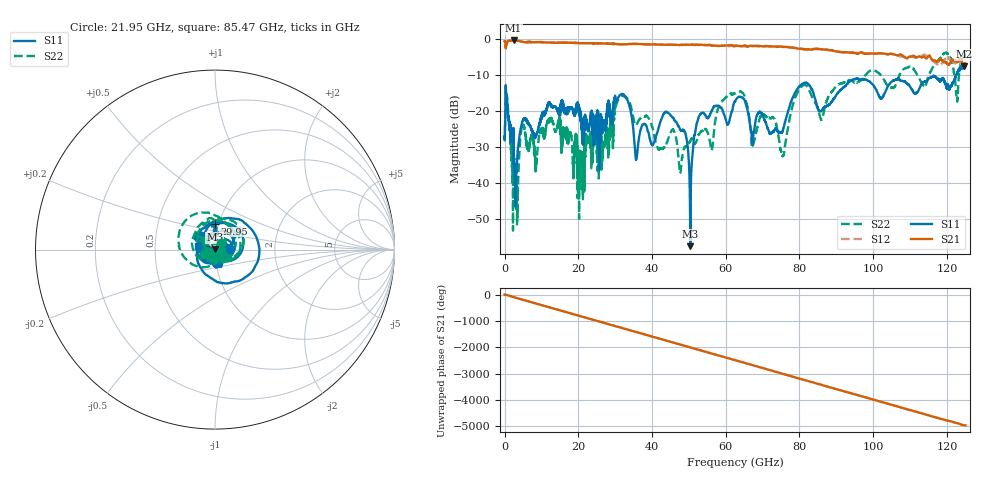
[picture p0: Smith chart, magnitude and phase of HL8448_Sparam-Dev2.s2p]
! 7/28/2025 10:33:41 AM
! H:\PROTOTYPE_DATA\110GHZ - KELVIN BT\7-28-25\4378.S2P
! CHANNEL.1
! TR.MEASUREMENT
! CORRECTED.DATA
! RF.CORRECTION: FULL.TWO.PORT.CAL.PORT.1.2
! AVERAGING: 1 PointByPoint
! IF.BANDWIDTH: 1KHZ
! SWEEPTYPE:  FREQ.SWEEP(Linear)
! Reference Plane Port Info
! PORT:  PORT1  PORT2
! DISTANCE:  0  m  0  m
! TIME:  0  s  0  s
! PHASE.OFFSET:  0 °  0 °
! LOSS:  0  dB  0  dB
! REF.LOSS:  0  dB  0  dB
! REF.FREQ:  0  Hz  0  Hz
! Power Info
! POWER:  -10  dBm  -10  dBm
! EFF.POWER:  -10  dBm  -10  dBm
! POWER(>54G):  -10  dBm  -10  dBm
! EFF.POWER(>54G):  -10  dBm  -10  dBm
! SOURCE.ATTEN:  0  dB  0  dB
! TEST.ATTEN:  0  dB  0  dB
# GHZ S RI R 50.0
! FREQ.GHZ  S11RE  S11IM  S21RE  S21IM  S12RE  S12IM  S22RE  S22IM
!; PortSelection: Port_12
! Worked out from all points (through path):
!   5000 points, 25 MHz to 125 GHz, reference 50 ohm
!   highest |S21| = -0.36 dB at 2.45 GHz (marker M1); lowest = -7.5 dB at 124.6 GHz (marker M2)
!   group delay of S21, straight-line fit = 111 ps
!   lowest |S11| = -57.7 dB at 50.4 GHz (marker M3), VSWR 1.00, Z = 49.9 + j0.101 ohm
!   |S11| at or under -10 dB: start of sweep to 122.5 GHz
!   |S22| runs from -53.3 to -3.8 dB; largest |S21 - S12| = 0.13
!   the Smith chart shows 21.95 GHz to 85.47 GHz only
!   S11 on the Smith chart (normalised r, x): 21.95 GHz: 1.18, +0.01; 29.95 GHz: 0.95, +0.28; 85.47 GHz: 0.82, +0.03
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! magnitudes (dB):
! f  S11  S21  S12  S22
! 25 MHz  -27.1  -0.6  -0.5  -27.3
! 875 MHz  -19.5  -0.6  -0.6  -18.7
! 2.45 GHz  -25.0  -0.4  -0.4  -27.1
! 12.38 GHz  -17.9  -0.9  -0.9  -23.0
! 20.88 GHz  -23.7  -1.1  -1.1  -32.7
! 21.95 GHz  -21.8  -1.1  -1.1  -26.4
! 29.95 GHz  -16.8  -1.3  -1.4  -19.6
! 33.27 GHz  -16.8  -1.4  -1.4  -16.5
! 35.75 GHz  -33.5  -1.3  -1.3  -23.9
! 41.7 GHz  -25.1  -1.5  -1.5  -30.5
! 48.7 GHz  -25.5  -1.6  -1.6  -30.4
! 50.4 GHz  -57.7  -1.5  -1.5  -28.4
! 53.08 GHz  -21.0  -1.5  -1.6  -26.0
! 62.52 GHz  -17.4  -1.9  -1.9  -15.1
! 75.38 GHz  -25.7  -2.1  -2.1  -32.3
! 79.47 GHz  -13.8  -2.6  -2.5  -14.9
! 83.35 GHz  -13.9  -2.9  -2.8  -15.9
! 85.47 GHz  -20.0  -2.8  -2.7  -21.3
! 104.2 GHz  -12.8  -4.2  -4.2  -13.1
! 122.7 GHz  -9.6  -6.3  -6.1  -16.3
! 124.6 GHz  -7.5  -7.5  -6.8  -4.7
! 125 GHz  -7.4  -6.8  -8.0  -4.4
